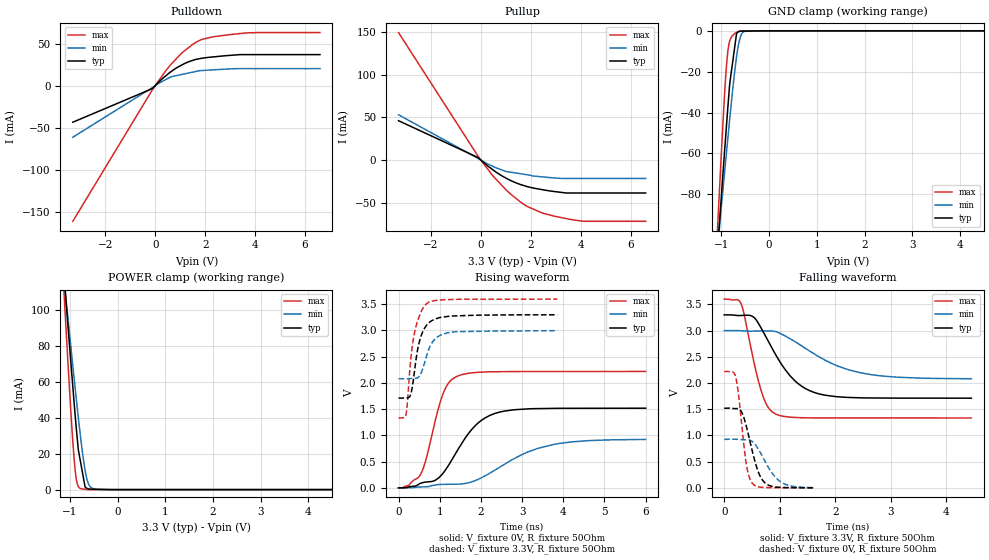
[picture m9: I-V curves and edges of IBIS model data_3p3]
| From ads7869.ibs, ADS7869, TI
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|   data_3p3 Model
[Model]   data_3p3
Model_type   I/O
Polarity   Non-Inverting
Enable   Active-Low
Vinl = 0.8
Vinh = 2.0
Vmeas = 1.65
Vref = 1.65
Cref = 30pF
Rref = 50
|   typ   min   max
|   (nom PVT)   (fast PVT)   (slow PVT)
|C_comp from frequency sweep method (F=8MHz)
|C_comp   3.291e-12   3.232e-12   3.482e-12
|ON state : BUFFER OUTPUT TURNED HIGH
|C_comp   3.511e-12   3.452e-12   3.655e-12
|OFF state: BUFFER OUTPUT TURNED LOW
|C_comp   3.130e-12   2.954e-12   3.310e-12
|C_comp from LC tank measurement(L=1nH)
|Resonant Frequency(Hz)   2.990e+09   3.030e+09   2.950e+09
C_comp   2.836e-12   2.762e-12   2.914e-12
|ON state : BUFFER OUTPUT TURNED HIGH
|Resonant Frequency(Hz)   2.990e+09   3.030e+09   2.950e+09
|C_comp   2.836e-12   2.762e-12   2.914e-12
|OFF state: BUFFER OUTPUT TURNED LOW
|Resonant Frequency(Hz)   2.920e+09   3.030e+09   2.820e+09
|C_comp   2.974e-12   2.762e-12   3.188e-12
| Where nom  PVT is Nominal Process, 3.3V, 36C
|   Fast PVT is Strong Process,  3.6V, -40C
|   Slow PVT is Weak Process,   3V, 96C
[Voltage Range]   3.3   3   3.6
|Ambient Temperature   25   85   -40
|Junction Temperature
[Temperature Range]   36   96   -40
[Pullup Reference]   3.3   3   3.6
[Pulldown Reference]   0   0   0
[Power Clamp Reference]   3.3   3   3.6
[GND Clamp Reference]   0   0   0
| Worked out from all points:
|   slope of the pulldown table from 0 to 0.495 V, typ, clamps not added: 36.8 ohm
|   slope of the pullup table from 0 to 0.495 V, typ, clamps not added: 42.5 ohm
|   GND clamp passes 1 mA (typ) near -0.67 V on its own axis
|   POWER clamp passes 1 mA (typ) near -0.66 V on its own axis
|   falling waveform, V_fixture 3.3V, R_fixture 50Ohm: 20-80 % time 588ps typ, 974ps min, 295ps max; typ from 3.3 V to 1.71 V
|   rising waveform, V_fixture 0V, R_fixture 50Ohm: 20-80 % time 797ps typ, 1.34ns min, 442ps max; typ from 0 V to 1.52 V
|   rising waveform, V_fixture 3.3V, R_fixture 50Ohm: 20-80 % time 235ps typ, 273ps min, 217ps max; typ from 1.71 V to 3.3 V
|   falling waveform, V_fixture 0V, R_fixture 50Ohm: 20-80 % time 225ps typ, 323ps min, 141ps max; typ from 1.52 V to 0.002 V
[Pulldown]
|   Voltage   I(typ)   I(min)   I(max)
-3.3V     -43.47mA   -61.36mA   -161.3mA
-118.8mV  -3.57mA    -2.371mA   -5.166mA
19.1fV    101uA      60.28uA    155.1uA
606mV     16.09mA    10.1mA     24.47mA
1.056V    24.44mA    13.29mA    38.48mA
1.546V    30.53mA    16.39mA    49.99mA
1.855V    32.58mA    17.97mA    54.84mA
2.248V    34mA       18.73mA    57.73mA
3.551V    36.96mA    20.26mA    62.5mA
6.6V      36.96mA    20.26mA    63.18mA
[GND Clamp]
|   Voltage   I(typ)   I(min)   I(max)
-3.3V     -837.3mA   -661mA     -1.124A
-1.231V   -156.2mA   -143.5mA   -165.8mA
-1.014V   -85.23mA   -89.4mA    -65.68mA
-924mV    -55.93mA   -67.06mA   -27.39mA
-895.2mV  -46.86mA   -60.04mA   -17.6mA
-859.2mV  -35.77mA   -51.26mA   -8.966mA
-825mV    -25.72mA   -42.91mA   -4.87mA
-683.1mV  -1.481mA   -12.72mA   -787.6uA
-643.2mV  -466.1uA   -6.971mA   -320.5uA
-558mV    -142.2uA   -932uA     -35.72uA
-354mV    -89.88uA   -1.244uA   0A
6.6V      0A         0A         0A
[Pullup]
|   Voltage   I(typ)   I(min)   I(max)
-3.3V     46.04mA    53mA       149.1mA
-118.8mV  3.039mA    2.048mA    4.774mA
19.1fV    -85.34uA   -51.72uA   -142.2uA
516mV     -12.1mA    -7.826mA   -19.59mA
1.009V    -21.09mA   -13.28mA   -34.89mA
1.574V    -28.47mA   -15.88mA   -48.81mA
1.855V    -30.99mA   -17.17mA   -54.19mA
2.42V     -34.37mA   -19.5mA    -61.41mA
3.409V    -38.43mA   -21.45mA   -68.31mA
3.691V    -38.43mA   -21.45mA   -69.84mA
4.138V    -38.43mA   -21.45mA   -71.54mA
6.6V      -38.43mA   -21.45mA   -71.54mA
[POWER Clamp]
|   Voltage   I(typ)   I(min)   I(max)
-3.3V     861.2mA    687.7mA    1.131A
-1.95V    400.6mA    333.3mA    495.5mA
-1.047V   92.47mA    96.3mA     72.62mA
-956.4mV  62.42mA    72.87mA    32.8mA
-884.4mV  39.15mA    54.55mA    9.09mA
-825mV    22.07mA    39.81mA    1.681mA
-762mV    12.9mA     25.58mA    437.8uA
-683.1mV  1.416mA    10.76mA    181.7uA
-627mV    551uA      4.198mA    5.339uA
-561mV    245.1uA    1.16mA     3.773uA
-420mV    167uA      103.9uA    427.2nA
6.6V      0A         0A         0A
[Ramp]
R_load = 50
|   typ   min   max
dV/dt_r   0.911132/7.97418e-10   0.554018/1.33556e-09   1.33129/4.42232e-10
dV/dt_f   0.953346/5.88191e-10   0.552493/9.77815e-10   1.36055/2.95269e-10
[Falling Waveform]
V_fixture = 3.3V
V_fixture_min = 3V
V_fixture_max = 3.6V
R_fixture = 50Ohm
|   Time   V(typ)   V(min)   V(max)
0s        3.3V       3V         3.6V
310.1ps   3.289V     2.996V     3.496V
527.4ps   3.257V     2.99V      2.438V
680.9ps   3.019V     2.993V     1.803V
802.9ps   2.78V      2.994V     1.519V
921.8ps   2.55V      2.983V     1.411V
1.306ns   2.011V     2.768V     1.342V
1.765ns   1.779V     2.467V     1.335V
2.654ns   1.715V     2.159V     1.334V
4.454ns   1.711V     2.081V     1.333V
[Rising Waveform]
V_fixture = 0V
V_fixture_min = 0V
V_fixture_max = 0V
R_fixture = 50Ohm
|   Time   V(typ)   V(min)   V(max)
0s        856pV      10.16nV    722.1pV
248.2ps   17.54mV    1.471mV    46.06mV
537.7ps   88.13mV    17.67mV    259.1mV
680.9ps   112mV      21.55mV    582.7mV
1.073ns   273.2mV    66.28mV    1.779V
1.399ns   672.5mV    70.33mV    2.118V
1.883ns   1.202V     146.1mV    2.2V
2.454ns   1.445V     392.7mV    2.215V
3.734ns   1.515V     822.8mV    2.218V
6ns       1.519V     923.4mV    2.219V
[Rising Waveform]
V_fixture = 3.3V
V_fixture_min = 3V
V_fixture_max = 3.6V
R_fixture = 50Ohm
|   Time   V(typ)   V(min)   V(max)
0s        1.711V     2.079V     1.332V
182.4ps   1.718V     2.079V     1.4V
290.4ps   1.769V     2.084V     2.394V
355.4ps   2.028V     2.088V     2.81V
428.5ps   2.464V     2.088V     3.092V
549.8ps   2.9V       2.191V     3.359V
695.9ps   3.114V     2.549V     3.52V
890.1ps   3.218V     2.841V     3.571V
1.258ns   3.274V     2.965V     3.591V
3.854ns   3.299V     2.997V     3.598V
[Falling Waveform]
V_fixture = 0V
V_fixture_min = 0V
V_fixture_max = 0V
R_fixture = 50Ohm
|   Time   V(typ)   V(min)   V(max)
0s        1.519V     926.2mV    2.219V
156.6ps   1.515V     928.3mV    2.212V
214ps     1.513V     928.1mV    2.081V
305.1ps   1.463V     921.5mV    1.313V
399.6ps   1.171V     918.3mV    444.9mV
509.6ps   685mV      881.8mV    83.12mV
630.6ps   261.5mV    711.9mV    17.14mV
770.3ps   67.25mV    438.3mV    6.427mV
1.065ns   8.44mV     85.75mV    1.966mV
1.619ns   1.846mV    6.601mV    1.034mV
